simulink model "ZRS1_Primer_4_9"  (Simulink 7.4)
settings: Solver=ode45  StartTime=0.0  StopTime=10.0  FixedStep=1.e-5  RelTol=1.e-3
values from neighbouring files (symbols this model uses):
  kp = 18    [ZRS1_Primer4_10_1.m]    (also in ZRS1_Primer4_10_2.m; ZRS1_Primer4_10_nih_preiz.m = 30; ZRS1_Primer4_9.m = 19; ZRS2_primer_3_9_a.m = 5.95662143529)
  motnja = 1    [ZRS1_Primer4_9.m]
  referenca = 1    [ZRS1_Primer4_10_1.m]    (also in ZRS1_Primer4_10_2.m; ZRS1_Primer4_10_nih_preiz.m; ZRS1_Primer4_9.m = 0)
  td = 0.351    [ZRS1_Primer4_10_1.m]    (also in ZRS1_Primer4_10_2.m = 0.7692; ZRS1_Primer4_10_nih_preiz.m = 0; ZRS1_Primer4_9.m = 0.210526315789)
  ti = 1.405    [ZRS1_Primer4_10_1.m]    (also in ZRS1_Primer4_10_2.m = 3.077; ZRS1_Primer4_10_nih_preiz.m = inf; ZRS1_Primer4_9.m = 2)

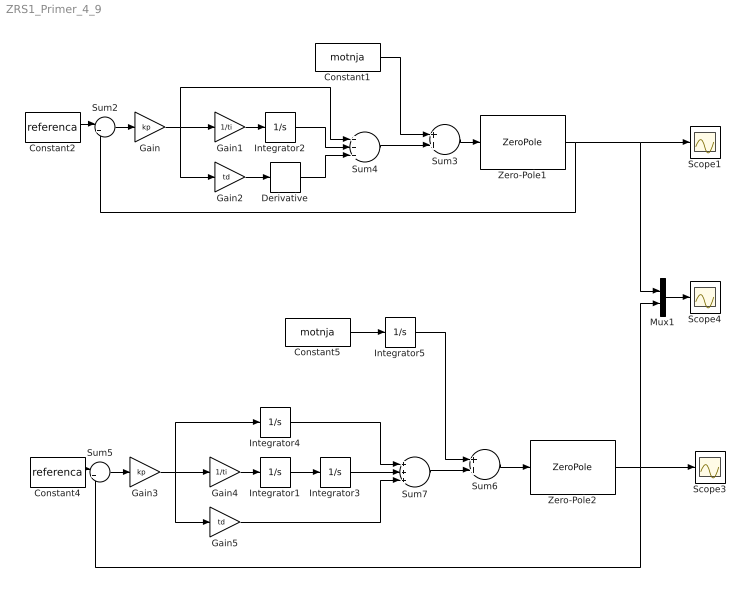
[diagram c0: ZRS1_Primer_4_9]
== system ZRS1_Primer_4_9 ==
  Constant1 : Constant  Value=motnja  OutDataType=sfix(16)  OutScaling=2^0
  Constant2 : Constant  Value=referenca  OutDataType=sfix(16)  OutScaling=2^0
  Constant4 : Constant  Value=referenca  OutDataType=sfix(16)  OutScaling=2^0
  Constant5 : Constant  Value=motnja  OutDataType=sfix(16)  OutScaling=2^0
  Derivative : Derivative
  Gain : Gain  Gain=kp  ParameterDataType=sfix(16)  ParameterScaling=2^0  OutDataType=sfix(16)  OutScaling=2^0
  Gain1 : Gain  Gain=1/ti  ParameterDataType=sfix(16)  ParameterScaling=2^0  OutDataType=sfix(16)  OutScaling=2^0
  Gain2 : Gain  Gain=td  ParameterDataType=sfix(16)  ParameterScaling=2^0  OutDataType=sfix(16)  OutScaling=2^0
  Gain3 : Gain  Gain=kp  ParameterDataType=sfix(16)  ParameterScaling=2^0  OutDataType=sfix(16)  OutScaling=2^0
  Gain4 : Gain  Gain=1/ti  ParameterDataType=sfix(16)  ParameterScaling=2^0  OutDataType=sfix(16)  OutScaling=2^0
  Gain5 : Gain  Gain=td  ParameterDataType=sfix(16)  ParameterScaling=2^0  OutDataType=sfix(16)  OutScaling=2^0
  Integrator{1..5} (5 alike) : Integrator
  Mux1 : Mux  Inputs=2
  Scope1 : Scope
  Scope3 : Scope
  Scope4 : Scope
  Sum2 : Sum  Inputs=|+-  OutDataType=sfix(16)  OutScaling=2^0
  Sum3 : Sum  OutDataType=sfix(16)  OutScaling=2^0
  Sum4 : Sum  Inputs=+++  OutDataType=sfix(16)  OutScaling=2^0
  Sum5 : Sum  Inputs=|+-  OutDataType=sfix(16)  OutScaling=2^0
  Sum6 : Sum  OutDataType=sfix(16)  OutScaling=2^0
  Sum7 : Sum  Inputs=+++  OutDataType=sfix(16)  OutScaling=2^0
  Zero-Pole1 : ZeroPole  Zeros=[]  Poles="[-1  -1/5]"  Gain=1/5
  Zero-Pole2 : ZeroPole  Zeros=[0]  Poles="[-1  -1/5]"  Gain=1/5
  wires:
  Constant2/1 -> Sum2/1
  Sum2/1 -> Gain/1
  Sum3/1 -> Zero-Pole1/1
  Zero-Pole1/1 -> Sum2/2, Scope1/1, Mux1/1
  Gain/1 -> Gain1/1, Sum4/1, Gain2/1
  Gain1/1 -> Integrator2/1
  Integrator2/1 -> Sum4/2
  Gain2/1 -> Derivative/1
  Derivative/1 -> Sum4/3
  Sum4/1 -> Sum3/2
  Constant4/1 -> Sum5/1
  Sum5/1 -> Gain3/1
  Sum6/1 -> Zero-Pole2/1
  Zero-Pole2/1 -> Sum5/2, Scope3/1, Mux1/2
  Gain3/1 -> Gain4/1, Gain5/1, Integrator4/1
  Gain4/1 -> Integrator1/1
  Sum7/1 -> Sum6/2
  Integrator1/1 -> Integrator3/1
  Integrator3/1 -> Sum7/2
  Integrator4/1 -> Sum7/1
  Gain5/1 -> Sum7/3
  Constant5/1 -> Integrator5/1
  Integrator5/1 -> Sum6/1
  Mux1/1 -> Scope4/1
  Constant1/1 -> Sum3/1
